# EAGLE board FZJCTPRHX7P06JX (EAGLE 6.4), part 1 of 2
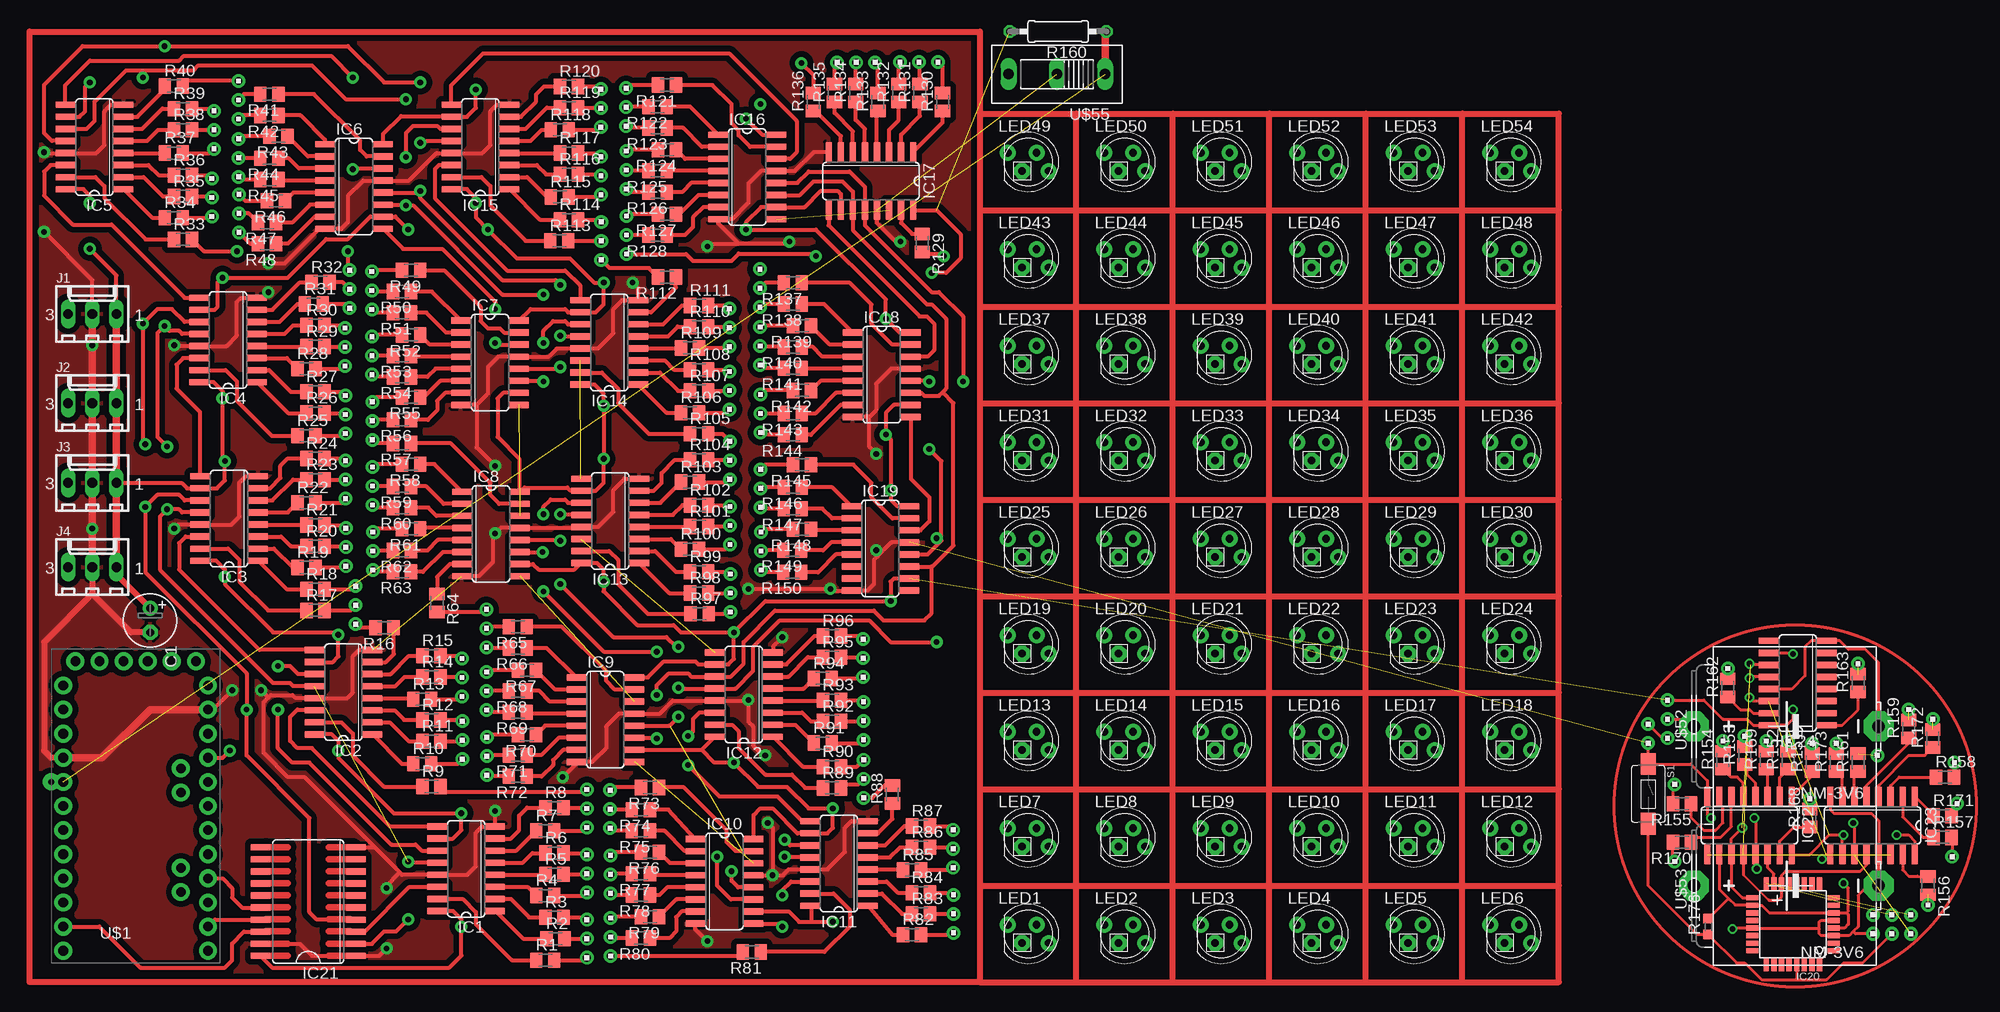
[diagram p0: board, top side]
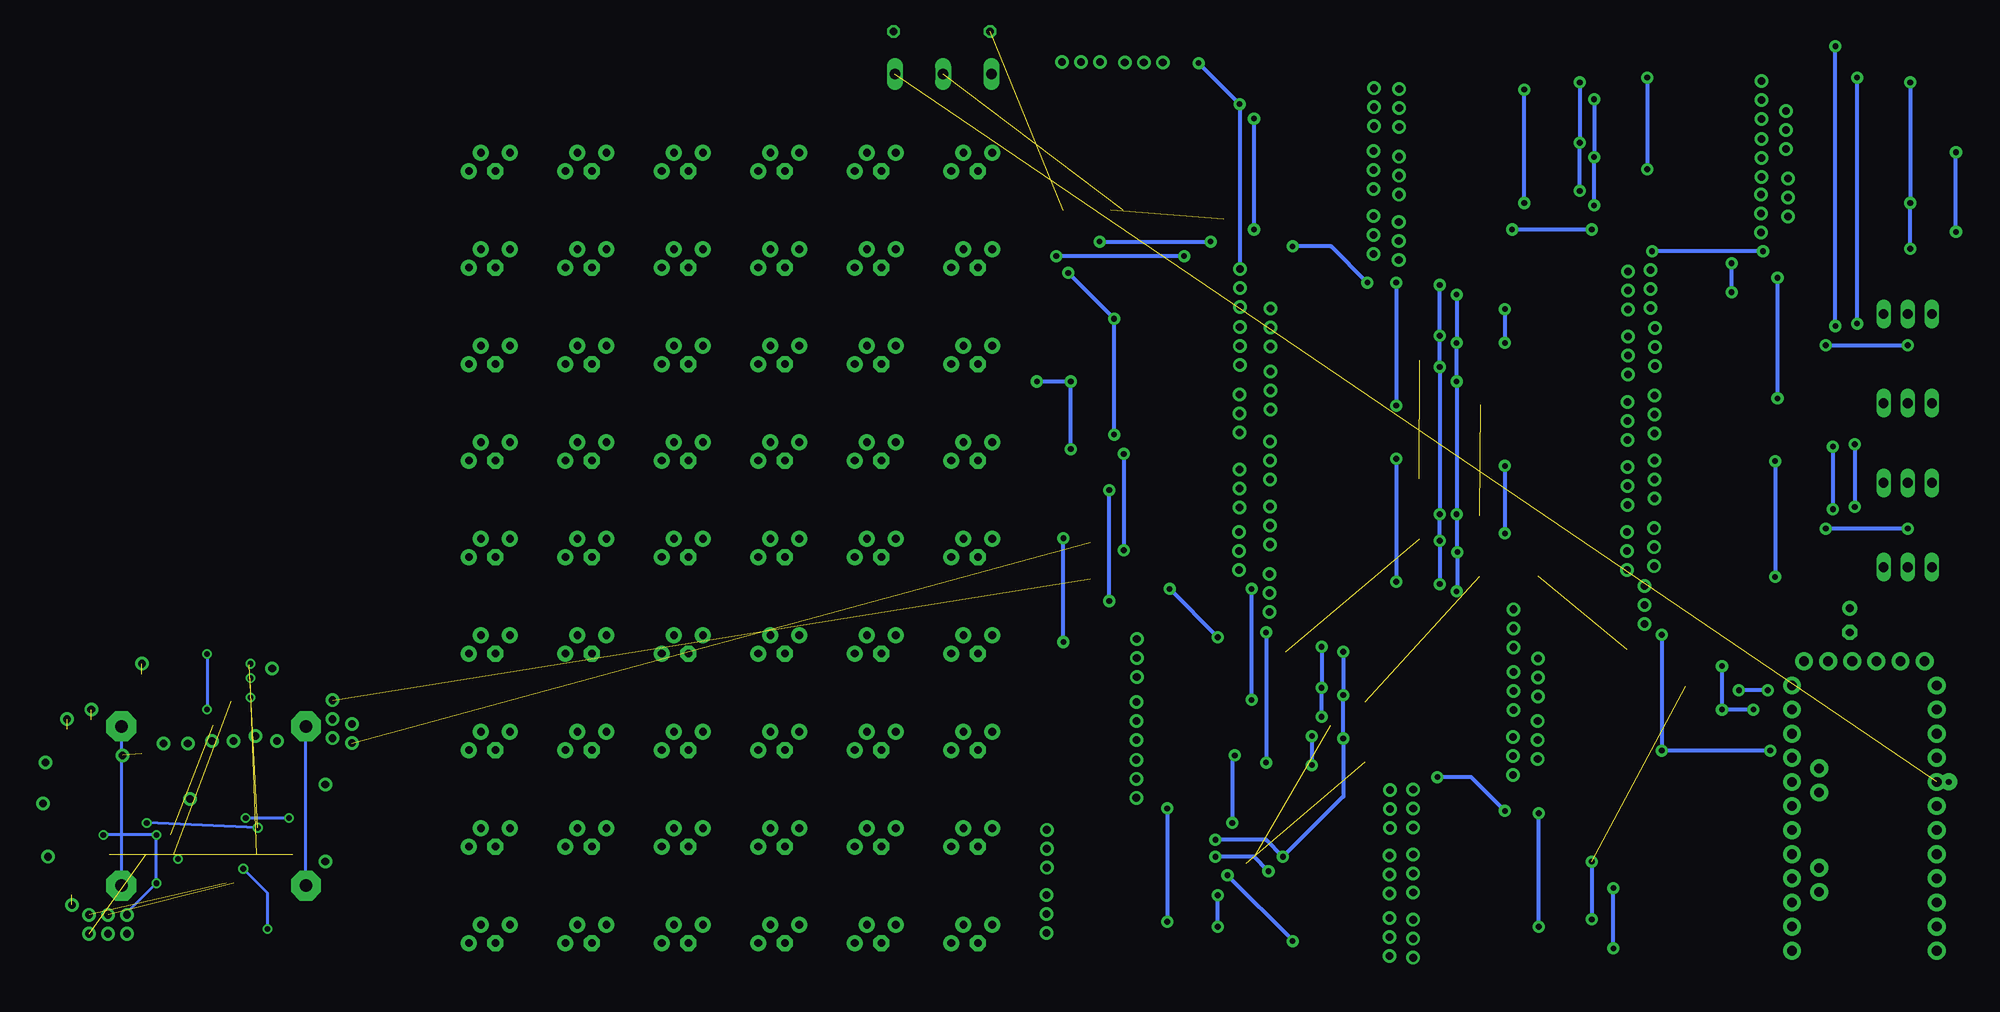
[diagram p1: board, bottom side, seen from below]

No outline drawn. Coordinates in mm, seen from the top.
Copper layers (1*16): Top 0.035mm / dielectric 1.5mm / Bottom 0.035mm
Design rules "default": minimum track width 10mil, minimum drill 24mil, track to track 8mil, track to pad 8mil, pad to pad 8mil, via to via 8mil, smd to smd 8mil, copper to edge 40mil, drill to drill 8mil, minimum pad ring 10mil, minimum via ring 8mil, stop-mask expansion 4mil, vias tented up to drill 0mil, thermal gap 10mil

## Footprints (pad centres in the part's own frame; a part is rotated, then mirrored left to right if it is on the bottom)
E2,5-6 = drill 0.813 pad 1.6: + -1.27,0 | drill 0.813 pad 1.6 octagon: - 1.27,0
SO16 = smd 0.66 x 2.032: 1 -4.445,-3.073; 2 -3.175,-3.073; 3 -1.905,-3.073; 4 -0.635,-3.073; 5 0.635,-3.073; 6 1.905,-3.073; 7 3.175,-3.073; 8 4.445,-3.073; 9 4.445,3.073; 10 3.175,3.073; 11 1.905,3.073; 12 0.635,3.073; 13 -0.635,3.073; 14 -1.905,3.073; 15 -3.175,3.073; 16 -4.445,3.073
TQFP32-08 = smd 1.27 x 0.559: 1 -4.293,2.8; 2 -4.293,2; 3 -4.293,1.2; 4 -4.293,0.4; 5 -4.293,-0.4; 6 -4.293,-1.2; 7 -4.293,-2; 8 -4.293,-2.8; 17 4.293,-2.8; 18 4.293,-2; 19 4.293,-1.2; 20 4.293,-0.4; 21 4.293,0.4; 22 4.293,1.2; 23 4.293,2; 24 4.293,2.8 | smd 0.559 x 1.27: 9 -2.8,-4.293; 10 -2,-4.293; 11 -1.2,-4.293; 12 -0.4,-4.293; 13 0.4,-4.293; 14 1.2,-4.293; 15 2,-4.293; 16 2.8,-4.293; 25 2.8,4.293; 26 2,4.293; 27 1.2,4.293; 28 0.4,4.293; 29 -0.4,4.293; 30 -1.2,4.293; 31 -2,4.293; 32 -2.8,4.293
SO20W = smd 0.66 x 2.032: 1 -5.715,-5.029; 2 -4.445,-5.029; 3 -3.175,-5.029; 4 -1.905,-5.029; 5 -0.635,-5.029; 6 0.635,-5.029; 7 1.905,-5.029; 8 3.175,-5.029; 9 4.445,-5.029; 10 5.715,-5.029; 11 5.715,5.029; 12 4.445,5.029; 13 3.175,5.029; 14 1.905,5.029; 15 0.635,5.029; 16 -0.635,5.029; 17 -1.905,5.029; 18 -3.175,5.029; 19 -4.445,5.029; 20 -5.715,5.029
6410-03 = drill 1.016 long: 1 2.54,0; 2 0,0; 3 -2.54,0
LED5MMRGB = drill 0.8 pad 1.676: 1 -2.159,0.968; 3 0.889,0.968; 4 2.159,-0.968 | drill 0.8 pad 1.676 octagon: 2 -0.635,-0.968
M0805 = smd 1.3 x 1.6: 1 -0.95,0; 2 0.95,0
0207/10 = drill 0.813 octagon: 1 -5.08,0; 2 5.08,0
R0603 = smd 1 x 1.1: 1 -0.85,0; 2 0.85,0
TACTILE-SWITCH-1101NE = smd 2.3 x 1.6: P$1 -3.15,0; P$2 3.15,0
ARDUINO_PRO_MINI = drill 1.016 pad 1.88: 1 -7.62,12.7; 2 -7.62,10.16; 3 -7.62,7.62; 4 -7.62,5.08; 5 -7.62,2.54; 6 -7.62,0; 7 -7.62,-2.54; 8 -7.62,-5.08; 9 -7.62,-7.62; 10 -7.62,-10.16; 11 -7.62,-12.7; 12 -7.62,-15.24; 13 7.62,-15.24; 14 7.62,-12.7; 15 7.62,-10.16; 16 7.62,-7.62; 17 7.62,-5.08; 18 7.62,-2.54; 19 7.62,0; 20 7.62,2.54; 21 7.62,5.08; 22 7.62,7.62; 23 7.62,10.16; 24 7.62,12.7; A4 4.763,1.429; A5 4.763,3.969; A6 4.763,-9.049; A7 4.763,-6.509; BLK -6.35,15.24; GND -3.81,15.24; GRN 6.35,15.24; RXI 1.27,15.24; TXO 3.81,15.24; VCC -1.27,15.24
1X3 = drill 0.8 pad 1.422: 1 -2,0; 2 0,0; 3 2,0
3.6V-NIMH-BATTERY = drill 1.321 pad 3.15 octagon: + -10.16,0; - 9.271,0
1X1 = drill 0.8 pad 1.422: 1 0,0
LIMIT-SWITCH = drill 1.118 long: 1 -5.08,0; 2 0,0; 3 5.08,0
2X3 = drill 0.8 pad 1.422: 1 -2,-1; 2 -2,1; 3 0,-1; 4 0,1; 5 2,-1; 6 2,1
1X2 = drill 0.8 pad 1.422: 1 -1,0; 2 1,0

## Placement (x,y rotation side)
C1  100uF  [E2,5-6]  12.7,38.1 270 top
IC1  74HC595D  [SO16]  45.97,11.94 90 top
IC2  74HC595D  [SO16]  33.05,30.53 90 top
IC3  74HC595D  [SO16]  21.01,48.82 90 top
IC4  74HC595D  [SO16]  20.9,67.61 90 top
IC5  74HC595D  [SO16]  6.83,87.93 90 top
IC6  74HC595D  [SO16]  34.16,83.77 270 top
IC7  74HC595D  [SO16]  48.49,65.23 270 top
IC8  74HC595D  [SO16]  48.59,47.19 270 top
IC9  74HC595D  [SO16]  60.63,27.64 270 top
IC10  74HC595D  [SO16]  73.18,10.62 270 top
IC11  74HC595D  [SO16]  85.22,12.5 90 top
IC12  74HC595D  [SO16]  75.21,30.28 90 top
IC13  74HC595D  [SO16]  61.14,48.56 90 top
IC14  74HC595D  [SO16]  61.04,67.36 90 top
IC15  74HC595D  [SO16]  47.47,87.93 90 top
IC16  74HC595D  [SO16]  75.56,84.79 270 top
IC17  74HC595D  [SO16]  88.6,84.35 180 top
IC18  74HC595D  [SO16]  89.74,63.96 270 top
IC19  74HC595D  [SO16]  89.59,45.67 270 top
IC20  MEGA8-AI  [TQFP32-08]  185.67,6.1 180 top
IC21  74LS245DW  [SO20W]  29.34,8.48 90 top
IC22  74HC595D  [SO16]  181.1,16.51 180 top
IC23  74HC595D  [SO16]  194.06,16.51 180 top
IC24  74HC595D  [SO16]  186.18,31.5 90 top
J1  22-27-2031-03  [6410-03]  6.6,70.36 0 top
J2  22-27-2031-03  [6410-03]  6.6,60.96 0 top
J3  22-27-2031-03  [6410-03]  6.6,52.58 0 top
J4  22-27-2031-03  [6410-03]  6.6,43.69 0 top
LED1  RGBLED_CA-5MM  [LED5MMRGB]  105.16,5.08 0 top
LED2  RGBLED_CA-5MM  [LED5MMRGB]  115.32,5.08 0 top
LED3  RGBLED_CA-5MM  [LED5MMRGB]  125.48,5.08 0 top
LED4  RGBLED_CA-5MM  [LED5MMRGB]  135.64,5.08 0 top
LED5  RGBLED_CA-5MM  [LED5MMRGB]  145.8,5.08 0 top
LED6  RGBLED_CA-5MM  [LED5MMRGB]  155.96,5.08 0 top
LED7  RGBLED_CA-5MM  [LED5MMRGB]  105.16,15.24 0 top
LED8  RGBLED_CA-5MM  [LED5MMRGB]  115.32,15.24 0 top
LED9  RGBLED_CA-5MM  [LED5MMRGB]  125.48,15.24 0 top
LED10  RGBLED_CA-5MM  [LED5MMRGB]  135.64,15.24 0 top
LED11  RGBLED_CA-5MM  [LED5MMRGB]  145.8,15.24 0 top
LED12  RGBLED_CA-5MM  [LED5MMRGB]  155.96,15.24 0 top
LED13  RGBLED_CA-5MM  [LED5MMRGB]  105.16,25.4 0 top
LED14  RGBLED_CA-5MM  [LED5MMRGB]  115.32,25.4 0 top
LED15  RGBLED_CA-5MM  [LED5MMRGB]  125.48,25.4 0 top
LED16  RGBLED_CA-5MM  [LED5MMRGB]  135.64,25.4 0 top
LED17  RGBLED_CA-5MM  [LED5MMRGB]  145.8,25.4 0 top
LED18  RGBLED_CA-5MM  [LED5MMRGB]  155.96,25.4 0 top
LED19  RGBLED_CA-5MM  [LED5MMRGB]  105.16,35.56 0 top
LED20  RGBLED_CA-5MM  [LED5MMRGB]  115.32,35.56 0 top
LED21  RGBLED_CA-5MM  [LED5MMRGB]  125.48,35.56 0 top
LED22  RGBLED_CA-5MM  [LED5MMRGB]  135.64,35.56 0 top
LED23  RGBLED_CA-5MM  [LED5MMRGB]  145.8,35.56 0 top
LED24  RGBLED_CA-5MM  [LED5MMRGB]  155.96,35.56 0 top
LED25  RGBLED_CA-5MM  [LED5MMRGB]  105.16,45.72 0 top
LED26  RGBLED_CA-5MM  [LED5MMRGB]  115.32,45.72 0 top
LED27  RGBLED_CA-5MM  [LED5MMRGB]  125.48,45.72 0 top
LED28  RGBLED_CA-5MM  [LED5MMRGB]  135.64,45.72 0 top
LED29  RGBLED_CA-5MM  [LED5MMRGB]  145.8,45.72 0 top
LED30  RGBLED_CA-5MM  [LED5MMRGB]  155.96,45.72 0 top
LED31  RGBLED_CA-5MM  [LED5MMRGB]  105.16,55.88 0 top
LED32  RGBLED_CA-5MM  [LED5MMRGB]  115.32,55.88 0 top
LED33  RGBLED_CA-5MM  [LED5MMRGB]  125.48,55.88 0 top
LED34  RGBLED_CA-5MM  [LED5MMRGB]  135.64,55.88 0 top
LED35  RGBLED_CA-5MM  [LED5MMRGB]  145.8,55.88 0 top
LED36  RGBLED_CA-5MM  [LED5MMRGB]  155.96,55.88 0 top
LED37  RGBLED_CA-5MM  [LED5MMRGB]  105.16,66.04 0 top
LED38  RGBLED_CA-5MM  [LED5MMRGB]  115.32,66.04 0 top
LED39  RGBLED_CA-5MM  [LED5MMRGB]  125.48,66.04 0 top
LED40  RGBLED_CA-5MM  [LED5MMRGB]  135.64,66.04 0 top
LED41  RGBLED_CA-5MM  [LED5MMRGB]  145.8,66.04 0 top
LED42  RGBLED_CA-5MM  [LED5MMRGB]  155.96,66.04 0 top
LED43  RGBLED_CA-5MM  [LED5MMRGB]  105.16,76.2 0 top
LED44  RGBLED_CA-5MM  [LED5MMRGB]  115.32,76.2 0 top
LED45  RGBLED_CA-5MM  [LED5MMRGB]  125.48,76.2 0 top
LED46  RGBLED_CA-5MM  [LED5MMRGB]  135.64,76.2 0 top
LED47  RGBLED_CA-5MM  [LED5MMRGB]  145.8,76.2 0 top
LED48  RGBLED_CA-5MM  [LED5MMRGB]  155.96,76.2 0 top
LED49  RGBLED_CA-5MM  [LED5MMRGB]  105.16,86.36 0 top
LED50  RGBLED_CA-5MM  [LED5MMRGB]  115.32,86.36 0 top
LED51  RGBLED_CA-5MM  [LED5MMRGB]  125.48,86.36 0 top
LED52  RGBLED_CA-5MM  [LED5MMRGB]  135.64,86.36 0 top
LED53  RGBLED_CA-5MM  [LED5MMRGB]  145.8,86.36 0 top
LED54  RGBLED_CA-5MM  [LED5MMRGB]  155.96,86.36 0 top
R1  150  [M0805]  54.31,2.31 0 top
R2  100  [M0805]  55.37,4.57 0 top
R3  100  [M0805]  55.27,6.83 0 top
R4  150  [M0805]  54.31,9.12 0 top
R5  100  [M0805]  55.27,11.35 0 top
R6  100  [M0805]  55.27,13.59 0 top
R7  150  [M0805]  54.31,15.93 0 top
R8  100  [M0805]  55.27,18.36 0 top
R9  100  [M0805]  42.32,20.6 0 top
R10  150  [M0805]  41.35,22.99 0 top
R11  100  [M0805]  42.32,25.37 0 top
R12  100  [M0805]  42.32,27.61 0 top
R13  150  [M0805]  41.35,29.79 0 top
R14  100  [M0805]  42.32,32.13 0 top
R15  100  [M0805]  42.32,34.37 0 top
R16  150  [M0805]  37.39,37.31 180 top
R17  100  [M0805]  30.12,39.14 0 top
R18  100  [M0805]  30.12,41.38 0 top
R19  150  [M0805]  29.16,43.66 0 top
R20  100  [M0805]  30.12,45.9 0 top
R21  100  [M0805]  30.12,48.13 0 top
R22  150  [M0805]  29.16,50.47 0 top
R23  100  [M0805]  30.12,52.91 0 top
R24  100  [M0805]  30.12,55.14 0 top
R25  150  [M0805]  29.16,57.53 0 top
R26  100  [M0805]  30.12,59.92 0 top
R27  100  [M0805]  30.12,62.15 0 top
R28  150  [M0805]  29.16,64.59 0 top
R29  100  [M0805]  30.12,66.93 0 top
R30  100  [M0805]  30.12,69.16 0 top
R31  150  [M0805]  29.92,71.4 0 top
R32  100  [M0805]  30.63,73.69 0 top
R33  100  [M0805]  16.15,78.21 0 top
R34  150  [M0805]  15.19,80.49 0 top
R35  100  [M0805]  16.15,82.73 0 top
R36  100  [M0805]  16.15,84.96 0 top
R37  150  [M0805]  15.19,87.3 0 top
R38  100  [M0805]  16.15,89.74 0 top
R39  100  [M0805]  16.15,91.97 0 top
R40  150  [M0805]  15.19,94.36 0 top
R41  100  [M0805]  25.25,93.5 180 top
R42  100  [M0805]  25.25,91.26 180 top
R43  150  [M0805]  26.21,89.08 180 top
R44  100  [M0805]  25.25,86.74 180 top
R45  100  [M0805]  25.25,84.51 180 top
R46  150  [M0805]  25.96,82.27 180 top
R47  100  [M0805]  24.99,79.98 180 top
R48  100  [M0805]  24.99,77.75 180 top
R49  150  [M0805]  40.18,74.96 180 top
R50  100  [M0805]  39.22,72.72 180 top
R51  100  [M0805]  39.22,70.48 180 top
R52  150  [M0805]  40.18,68.15 180 top
R53  100  [M0805]  39.22,65.96 180 top
R54  100  [M0805]  39.22,63.73 180 top
R55  150  [M0805]  40.18,61.59 180 top
R56  100  [M0805]  39.22,59.21 180 top
R57  100  [M0805]  39.22,56.72 180 top
R58  150  [M0805]  40.18,54.53 180 top
R59  100  [M0805]  39.22,52.2 180 top
R60  100  [M0805]  39.22,49.96 180 top
R61  150  [M0805]  40.18,47.73 180 top
R62  100  [M0805]  39.22,45.44 180 top
R63  100  [M0805]  39.22,43.21 180 top
R64  150  [M0805]  42.9,39.93 270 top
R65  100  [M0805]  51.41,37.41 180 top
R66  100  [M0805]  51.41,35.18 180 top
R67  150  [M0805]  52.37,32.84 180 top
R68  100  [M0805]  51.41,30.66 180 top
R69  100  [M0805]  51.41,28.42 180 top
R70  150  [M0805]  52.37,26.04 180 top
R71  100  [M0805]  51.41,23.9 180 top
R72  100  [M0805]  51.41,21.67 180 top
R73  150  [M0805]  65.33,20.5 180 top
R74  100  [M0805]  64.36,18.16 180 top
R75  100  [M0805]  64.36,15.93 180 top
R76  150  [M0805]  65.33,13.69 180 top
R77  100  [M0805]  64.36,11.4 180 top
R78  100  [M0805]  64.36,9.17 180 top
R79  150  [M0805]  65.33,6.88 180 top
R80  100  [M0805]  64.36,4.65 180 top
R81  100  [M0805]  76.05,3.17 180 top
R82  150  [M0805]  92.91,5 0 top
R83  100  [M0805]  93.88,7.19 0 top
R84  100  [M0805]  93.88,9.42 0 top
R85  150  [M0805]  92.91,11.81 0 top
R86  100  [M0805]  93.88,14.2 0 top
R87  100  [M0805]  93.88,16.43 0 top
R88  150  [M0805]  90.86,19.76 90 top
R89  100  [M0805]  84.48,20.45 0 top
R90  100  [M0805]  84.48,22.68 0 top
R91  150  [M0805]  83.52,25.17 0 top
R92  100  [M0805]  84.48,27.46 0 top
R93  100  [M0805]  84.48,29.69 0 top
R94  150  [M0805]  83.52,31.98 0 top
R95  100  [M0805]  84.48,34.21 0 top
R96  100  [M0805]  84.48,36.45 0 top
R97  150  [M0805]  70.56,38.79 0 top
R98  100  [M0805]  70.51,40.97 0 top
R99  100  [M0805]  70.51,43.21 0 top
R100  150  [M0805]  69.55,45.59 0 top
R101  100  [M0805]  70.51,47.98 0 top
R102  100  [M0805]  70.51,50.22 0 top
R103  150  [M0805]  69.55,52.65 0 top
R104  100  [M0805]  70.51,54.99 0 top
R105  100  [M0805]  70.51,57.73 0 top
R106  150  [M0805]  69.55,59.97 0 top
R107  100  [M0805]  70.51,62.26 0 top
R108  100  [M0805]  70.51,64.49 0 top
R109  150  [M0805]  69.55,66.78 0 top
R110  100  [M0805]  70.51,69.01 0 top
R111  100  [M0805]  70.51,71.25 0 top
R112  150  [M0805]  67.11,74.24 180 top
R113  100  [M0805]  55.78,78.05 0 top
R114  100  [M0805]  56.79,80.29 0 top
R115  150  [M0805]  55.83,82.68 0 top
R116  100  [M0805]  56.79,85.06 0 top
R117  100  [M0805]  56.79,87.3 0 top
R118  150  [M0805]  55.83,89.74 0 top
R119  100  [M0805]  56.79,92.08 0 top
R120  100  [M0805]  56.79,94.31 0 top
R121  150  [M0805]  67.11,94.46 180 top
R122  100  [M0805]  66.14,92.18 180 top
R123  100  [M0805]  66.14,89.94 180 top
R124  150  [M0805]  67.11,87.66 180 top
R125  100  [M0805]  66.14,85.42 180 top
R126  100  [M0805]  66.14,83.19 180 top
R127  150  [M0805]  67.11,80.85 180 top
R128  100  [M0805]  66.14,78.66 180 top
R129  100  [M0805]  94.01,77.83 270 top
R130  150  [M0805]  96.14,92.66 90 top
R131  100  [M0805]  93.75,93.62 90 top
R132  100  [M0805]  91.52,93.62 90 top
R133  150  [M0805]  89.33,92.66 90 top
R134  100  [M0805]  87,93.62 90 top
R135  100  [M0805]  84.76,93.62 90 top
R136  150  [M0805]  82.52,92.66 90 top
R137  100  [M0805]  80.37,73.63 180 top
R138  100  [M0805]  80.37,71.4 180 top
R139  150  [M0805]  81.33,69.11 180 top
R140  100  [M0805]  80.37,66.88 180 top
R141  100  [M0805]  80.37,64.64 180 top
R142  150  [M0805]  81.33,62.31 180 top
R143  100  [M0805]  80.37,59.87 180 top
R144  100  [M0805]  80.37,57.63 180 top
R145  150  [M0805]  81.33,54.48 180 top
R146  100  [M0805]  80.37,52.1 180 top
R147  100  [M0805]  80.37,49.86 180 top
R148  150  [M0805]  81.33,47.68 180 top
R149  100  [M0805]  80.31,45.49 180 top
R150  100  [M0805]  80.31,43.15 180 top
R151  100  [M0805]  187.71,23.11 90 top
R152  100  [M0805]  185.17,23.37 90 top
R153  100  [M0805]  180.59,23.88 90 top
R154  100  [M0805]  178.31,23.37 90 top
R155  100  [M0805]  173.99,18.8 180 top
R156  100  [M0805]  199.9,10.16 270 top
R157  100  [M0805]  201.42,15.24 0 top
R158  100  [M0805]  201.68,21.59 0 top
R159  100  [M0805]  197.87,26.67 90 top
R160  10K  [0207/10]  108.31,100.1 180 top
R161  100  [M0805]  192.53,23.11 90 top
R162  100  [M0805]  178.82,30.99 90 top
R163  100  [M0805]  192.53,31.5 90 top
R168  150  [M0805]  187.45,17.27 90 top
R169  150  [M0805]  182.88,23.37 90 top
R170  150  [M0805]  173.99,14.73 180 top
R171  150  [M0805]  201.42,17.53 0 top
R172  150  [M0805]  200.41,25.65 90 top
R173  150  [M0805]  190.25,23.11 90 top
R176  10K  [R0603]  176.78,5.84 90 top
S1  SWITCH-MOMENTARY-2-SMD-1101NE  [TACTILE-SWITCH-1101NE]  170.43,19.81 270 top
U$1  ARDUINO_PRO_MINI  [ARDUINO_PRO_MINI]  11.18,18.54 0 top
U$2  1X3  [1X3]  58.67,4.57 270 top
U$3  1X3  [1X3]  58.67,11.43 270 top
U$4  1X3  [1X3]  58.67,18.29 270 top
U$5  1X3  [1X3]  45.57,25.48 270 top
U$6  1X3  [1X3]  45.54,32.08 270 top
U$7  1X3  [1X3]  34.34,39.7 270 top
U$8  1X3  [1X3]  33.3,45.8 270 top
U$9  1X3  [1X3]  33.27,52.91 270 top
U$10  1X3  [1X3]  33.25,59.77 270 top
U$11  1X3  [1X3]  33.22,66.88 270 top
U$12  1X3  [1X3]  33.71,72.97 270 top
U$13  1X3  [1X3]  19.2,82.63 270 top
U$14  1X3  [1X3]  19.43,89.74 270 top
U$15  1X3  [1X3]  22,92.89 90 top
U$16  1X3  [1X3]  22.02,86.79 90 top
U$17  1X3  [1X3]  22.05,80.95 90 top
U$18  1X3  [1X3]  36.04,72.82 90 top
U$19  1X3  [1X3]  36.07,65.96 90 top
U$20  1X3  [1X3]  36.09,59.11 90 top
U$21  1X3  [1X3]  36.12,52.25 90 top
U$22  1X3  [1X3]  36.14,45.39 90 top
U$23  1X3  [1X3]  48.11,37.26 90 top
U$24  1X3  [1X3]  48.13,30.66 90 top
U$25  1X3  [1X3]  48.16,23.8 90 top
U$26  1X3  [1X3]  61.14,18.21 90 top
U$27  1X3  [1X3]  61.16,11.35 90 top
U$28  1X3  [1X3]  61.19,4.75 90 top
U$29  1X3  [1X3]  97.28,7.19 270 top
U$30  1X3  [1X3]  97.26,14.05 270 top
U$31  1X3  [1X3]  87.83,21.41 270 top
U$32  1X3  [1X3]  87.81,27.51 270 top
U$33  1X3  [1X3]  87.78,34.11 270 top
U$34  1X3  [1X3]  73.79,40.97 270 top
U$35  1X3  [1X3]  73.76,48.08 270 top
U$36  1X3  [1X3]  73.74,54.94 270 top
U$37  1X3  [1X3]  73.71,62.31 270 top
U$38  1X3  [1X3]  73.69,68.91 270 top
U$39  1X3  [1X3]  60.2,78.05 270 top
U$40  1X3  [1X3]  60.17,84.91 270 top
U$41  1X3  [1X3]  60.15,92.02 270 top
U$42  1X3  [1X3]  62.81,92.13 90 top
U$43  1X3  [1X3]  62.84,85.52 90 top
U$44  1X3  [1X3]  62.87,78.66 90 top
U$45  1X3  [1X3]  93.65,96.88 0 top
U$46  1X3  [1X3]  87.05,96.85 0 top
U$47  1X3  [1X3]  76.91,73.08 90 top
U$48  1X3  [1X3]  76.94,66.98 90 top
U$49  1X3  [1X3]  76.96,59.87 90 top
U$50  1X3  [1X3]  76.99,51.99 90 top
U$51  1X3  [1X3]  77.01,45.39 90 top
U$52  3.6V-NIMH-BATTERY  [3.6V-NIMH-BATTERY]  185.42,26.92 0 top
U$53  3.6V-NIMH-BATTERY  [3.6V-NIMH-BATTERY]  185.42,10.16 0 top
U$54  1X1  [1X1]  187.45,19.3 0 top
U$55  LIMIT-SWITCH  [LIMIT-SWITCH]  108.18,95.61 180 top
U$56  1X1  [1X1]  187.71,25.15 0 top
U$57  1X1  [1X1]  185.17,25.4 0 top
U$58  1X1  [1X1]  182.88,25.4 0 top
U$59  1X1  [1X1]  180.59,25.91 0 top
U$60  1X1  [1X1]  178.31,25.4 0 top
U$61  1X1  [1X1]  173.23,12.7 0 top
U$62  1X1  [1X1]  173.23,20.83 0 top
U$63  2X3  [2X3]  196.09,6.1 0 top
U$64  1X3  [1X3]  172.47,27.69 90 top
U$65  1X1  [1X1]  199.9,8.13 0 top
U$66  1X1  [1X1]  202.95,18.8 0 top
U$67  1X1  [1X1]  202.44,13.21 0 top
U$68  1X1  [1X1]  202.69,23.11 0 top
U$69  1X1  [1X1]  200.41,27.69 0 top
U$70  1X1  [1X1]  197.87,28.7 0 top
U$71  1X1  [1X1]  194.56,23.88 0 top
U$72  1X1  [1X1]  190.25,25.15 0 top
U$73  1X1  [1X1]  178.82,33.02 0 top
U$74  1X1  [1X1]  192.53,33.53 0 top
U$75  1X2  [1X2]  170.43,26.16 90 top

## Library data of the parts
C1 R1-R163 R168-R173 R176 = resistor
IC1-IC19 IC22-IC24 = 74xx-eu
IC20 = atmel; MPN: ATMEGA8-16AU; OC_FARNELL: 9171371; OC_NEWARK: 73M8863
IC21 = 74xx-us
J1-J4 = con-molex; OC_FARNELL: unknown; OC_NEWARK: unknown
LED1-LED54 = adafruit
S1 = SparkFun-Electromechanical
U$1 = SparkFun-Boards
U$2-U$51 U$54 U$56-U$75 = headers(2mm)
U$52 U$53 U$55 = ggaqquay

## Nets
CLOCK: IC1.11 IC2.11 IC3.11 IC4.11 IC5.11 IC6.11 IC7.11 IC8.11 IC9.11 IC10.11 IC11.11 IC12.11 IC13.11 IC14.11 IC15.11 IC16.11 IC17.11 IC18.11 IC19.11 IC21.4
CLOCK2: IC20.17 IC22.11 IC23.11 IC24.11 U$63.5
D8: IC21.18 U$1.11
D11: IC21.17 U$1.14
D13: IC21.16 U$1.16
DATA: IC1.14 IC21.3
DATA2: IC20.15 IC22.14 U$63.6
GND: C1.- IC1.8 IC1.13 IC2.8 IC2.13 IC3.8 IC3.13 IC4.8 IC4.13 IC5.8 IC5.13 IC6.8 IC6.13 IC7.8 IC7.13 IC8.8 IC8.13 IC9.8 IC9.13 IC10.8 IC10.13 IC11.8 IC11.13 IC12.8 IC12.13 IC13.8 IC13.13 IC14.8 IC14.13 IC15.8 IC15.13 IC16.8 IC16.13 IC17.8 IC17.13 IC18.8 IC18.13 IC19.8 IC19.13 IC20.3 IC20.5 IC20.21 IC21.1 IC21.10 IC21.19 IC22.8 IC22.13 IC23.8 IC23.13 IC24.8 IC24.13 J1.2 J2.2 J3.2 J4.2 S1.P$1 U$1.4 U$1.23 U$52.- U$53.- U$55.2 U$63.1 U$75.1
LATCH: IC1.12 IC2.12 IC3.12 IC4.12 IC5.12 IC6.12 IC7.12 IC8.12 IC9.12 IC10.12 IC11.12 IC12.12 IC13.12 IC14.12 IC15.12 IC16.12 IC17.12 IC18.12 IC19.12 IC21.2
LATCH2: IC20.14 IC22.12 IC23.12 IC24.12
MISO: IC20.16 U$63.4
N$1: R160.1 U$1.5 U$55.1
N$4: IC22.15 R168.1
N$5: R81.2 U$28.1
N$6: IC10.9 IC11.14
N$7: IC22.1 R151.1
N$8: IC22.2 R152.1
N$9: R168.2 U$54.1
N$10: R151.2 U$56.1
N$11: R152.2 U$57.1
N$12: R169.2 U$58.1
N$13: R153.2 U$59.1
N$14: R154.2 U$60.1
N$15: R170.2 U$61.1
N$16: R155.2 U$62.1
N$17: IC22.3 R169.1
N$18: IC22.4 R153.1
N$19: IC22.5 R154.1
N$20: IC22.6 R170.1
N$21: IC22.7 R155.1
N$22: IC23.15 R156.1
N$23: R156.2 U$65.1
N$24: R171.2 U$66.1
N$25: R157.2 U$67.1
N$26: R158.2 U$68.1
N$27: R172.2 U$69.1
N$28: R159.2 U$70.1
N$29: IC1.15 R1.1
N$30: IC1.1 R2.1
N$31: IC1.2 R3.1
N$32: R1.2 U$2.3
N$33: R2.2 U$2.2
N$34: R3.2 U$2.1
N$35: R4.2 U$3.3
N$36: R5.2 U$3.2
N$37: R6.2 U$3.1
N$38: R7.2 U$4.3
N$39: R8.2 U$4.2
N$40: IC1.3 R4.1
N$41: IC1.4 R5.1
N$42: IC1.5 R6.1
N$43: IC1.6 R7.1
N$44: IC1.7 R8.1
N$45: IC2.15 R9.1
N$46: R9.2 U$4.1
N$47: R10.2 U$5.3
N$48: R11.2 U$5.2
N$49: R12.2 U$5.1
N$50: R13.2 U$6.3
N$51: R14.2 U$6.2
N$52: R15.2 U$6.1
N$53: R16.2 U$7.3
N$54: R17.2 U$7.2
N$55: R18.2 U$7.1
N$56: R19.2 U$8.3
N$57: R20.2 U$8.2
N$58: R21.2 U$8.1
N$59: R22.2 U$9.3
N$60: R23.2 U$9.2
N$61: R24.2 U$9.1
N$62: R25.2 U$10.3
N$63: R26.2 U$10.2
N$64: R27.2 U$10.1
N$65: R28.2 U$11.3
N$66: R29.2 U$11.2
N$67: R30.2 U$11.1
N$68: R31.2 U$12.3
N$69: R32.2 U$12.2
N$70: R33.2 U$12.1
N$71: R34.2 U$13.3
N$72: R35.2 U$13.2
N$73: R36.2 U$13.1
N$74: R37.2 U$14.3
N$75: R38.2 U$14.2
N$76: R39.2 U$14.1
N$77: R40.2 U$15.3
N$78: R41.2 U$15.2
N$79: R42.2 U$15.1
N$80: R43.2 U$16.3
N$81: R44.2 U$16.2
N$82: R45.2 U$16.1
N$83: R46.2 U$17.3
N$84: R47.2 U$17.2
N$85: R48.2 U$17.1
N$86: R49.2 U$18.3
N$87: R50.2 U$18.2
N$88: R51.2 U$18.1
N$89: R52.2 U$19.3
N$90: R53.2 U$19.2
N$91: R54.2 U$19.1
N$92: R55.2 U$20.3
N$93: R56.2 U$20.2
N$94: R57.2 U$20.1
N$95: R58.2 U$21.3
N$96: R59.2 U$21.2
N$97: R60.2 U$21.1
N$98: R61.2 U$22.3
N$99: R62.2 U$22.2
N$100: R63.2 U$22.1
N$101: R64.2 U$23.3
N$102: R65.2 U$23.2
N$103: R66.2 U$23.1
N$104: R67.2 U$24.3
N$105: R68.2 U$24.2
N$106: R69.2 U$24.1
N$107: R70.2 U$25.3
N$108: R71.2 U$25.2
N$109: R72.2 U$25.1
N$110: R73.2 U$26.3
N$111: R74.2 U$26.2
N$112: R75.2 U$26.1
N$113: R76.2 U$27.3
N$114: R77.2 U$27.2
N$115: R78.2 U$27.1
N$116: R79.2 U$28.3
N$117: R80.2 U$28.2
N$118: R82.2 U$29.3
N$119: R83.2 U$29.2
N$120: R84.2 U$29.1
N$121: R85.2 U$30.3
N$122: R86.2 U$30.2
N$123: R87.2 U$30.1
N$124: R88.2 U$31.3
N$125: R89.2 U$31.2
N$126: R90.2 U$31.1
N$127: R91.2 U$32.3
N$128: R92.2 U$32.2
N$129: R93.2 U$32.1
N$130: R94.2 U$33.3
N$131: R95.2 U$33.2
N$132: R96.2 U$33.1
N$133: R97.2 U$34.3
N$134: R98.2 U$34.2
N$135: R99.2 U$34.1
N$136: R100.2 U$35.3
N$137: R101.2 U$35.2
N$138: R102.2 U$35.1
N$139: R103.2 U$36.3
N$140: R104.2 U$36.2
N$141: R105.2 U$36.1
N$142: R106.2 U$37.3
N$143: R107.2 U$37.2
N$144: R108.2 U$37.1
N$145: R109.2 U$38.3
N$146: R110.2 U$38.2
N$147: R111.2 U$38.1
N$148: R112.2 U$39.3
N$149: R113.2 U$39.2
N$150: R114.2 U$39.1
N$151: R115.2 U$40.3
N$152: R116.2 U$40.2
N$153: R117.2 U$40.1
N$154: R118.2 U$41.3
N$155: R119.2 U$41.2
N$156: R120.2 U$41.1
N$157: R121.2 U$42.3
N$158: R122.2 U$42.2
N$159: R123.2 U$42.1
N$160: R124.2 U$43.3
N$161: R125.2 U$43.2
N$162: R126.2 U$43.1
N$163: R127.2 U$44.3
N$164: R128.2 U$44.2
N$165: R129.2 U$44.1
N$166: R130.2 U$45.3
N$167: R131.2 U$45.2
N$168: R132.2 U$45.1
N$169: R133.2 U$46.3
N$170: R134.2 U$46.2
N$171: R135.2 U$46.1
N$172: R136.2 U$47.3
N$173: R137.2 U$47.2
N$174: R138.2 U$47.1
N$175: R139.2 U$48.3
N$176: R140.2 U$48.2
N$177: R141.2 U$48.1
N$178: R142.2 U$49.3
N$179: R143.2 U$49.2
N$180: R144.2 U$49.1
N$181: R145.2 U$50.3
N$182: R146.2 U$50.2
N$183: R147.2 U$50.1
N$184: R148.2 U$51.3
N$185: R149.2 U$51.2
N$186: R150.2 U$51.1
N$187: R161.2 U$71.1
N$188: R173.2 U$72.1
N$189: R162.2 U$73.1
N$190: R163.2 U$74.1
N$196: IC11.15 R81.1
N$197: IC11.1 R82.1
N$198: IC11.2 R83.1
N$199: IC11.3 R84.1
N$200: IC11.4 R85.1
N$201: IC11.5 R86.1
N$202: IC11.6 R87.1
N$203: IC11.7 R88.1
N$204: IC12.15 R89.1
N$205: IC12.1 R90.1
N$206: IC12.2 R91.1
N$207: IC12.3 R92.1
N$208: IC12.4 R93.1
N$209: IC12.5 R94.1
N$210: IC12.6 R95.1
N$211: IC12.7 R96.1
N$212: IC13.15 R97.1
N$213: IC13.1 R98.1
N$214: IC13.2 R99.1
N$215: IC13.3 R100.1
N$216: IC13.4 R101.1
N$217: IC13.5 R102.1
N$218: IC13.6 R103.1
N$219: IC13.7 R104.1
N$220: IC14.15 R105.1
N$221: IC14.1 R106.1
N$222: IC14.2 R107.1
N$223: IC14.3 R108.1
N$224: IC14.4 R109.1
N$225: IC14.5 R110.1
N$226: IC14.6 R111.1
N$227: IC14.7 R112.1
N$228: IC15.15 R113.1
N$229: IC15.1 R114.1
N$230: IC15.2 R115.1
N$231: IC15.3 R116.1
N$232: IC15.4 R117.1
N$233: IC15.5 R118.1
N$234: IC15.6 R119.1
N$235: IC15.7 R120.1
N$236: IC16.15 R121.1
N$237: IC16.1 R122.1
N$238: IC16.2 R123.1
N$239: IC16.3 R124.1
N$240: IC16.4 R125.1
N$241: IC16.5 R126.1
N$242: IC16.6 R127.1
N$243: IC16.7 R128.1
N$244: IC17.15 R129.1
N$245: IC17.1 R130.1
N$246: IC17.2 R131.1
N$247: IC17.3 R132.1
N$248: IC17.4 R133.1
N$249: IC17.5 R134.1
N$250: IC17.6 R135.1
N$251: IC17.7 R136.1
N$252: IC18.15 R137.1
N$253: IC18.1 R138.1
N$254: IC18.2 R139.1
N$255: IC18.3 R140.1
N$256: IC18.4 R141.1
N$257: IC18.5 R142.1
N$258: IC18.6 R143.1
N$259: IC18.7 R144.1
N$260: IC19.15 R145.1
N$261: IC19.1 R146.1
N$262: IC19.2 R147.1
N$263: IC19.3 R148.1
N$264: IC19.4 R149.1
N$265: IC19.5 R150.1
N$273: IC24.1 R163.1
N$274: IC24.15 R162.1
N$275: IC23.7 R173.1
N$276: IC10.7 R80.1
N$277: IC10.6 R79.1
N$278: IC10.5 R78.1
N$279: IC10.4 R77.1
N$280: IC10.3 R76.1
N$281: IC10.2 R75.1
N$282: IC10.1 R74.1
N$283: IC10.15 R73.1
N$284: IC9.7 R72.1
N$285: IC9.6 R71.1
N$286: IC9.5 R70.1
N$287: IC9.4 R69.1
N$288: IC9.3 R68.1
N$289: IC9.2 R67.1
N$290: IC9.1 R66.1
N$291: IC9.15 R65.1
N$292: IC8.7 R64.1
N$293: IC8.6 R63.1
N$294: IC8.5 R62.1
N$295: IC8.4 R61.1
N$296: IC8.3 R60.1
N$297: IC8.2 R59.1
N$298: IC8.1 R58.1
N$299: IC8.15 R57.1
N$300: IC7.7 R56.1
N$301: IC7.6 R55.1
N$302: IC7.5 R54.1
N$303: IC7.4 R53.1
N$304: IC7.3 R52.1
N$305: IC7.2 R51.1
N$306: IC7.1 R50.1
N$307: IC7.15 R49.1
N$308: IC6.7 R48.1
N$309: IC6.6 R47.1
N$310: IC6.5 R46.1
N$311: IC6.4 R45.1
N$312: IC6.3 R44.1
N$313: IC6.2 R43.1
N$314: IC6.1 R42.1
N$315: IC6.15 R41.1
N$316: IC5.7 R40.1
N$317: IC5.6 R39.1
N$318: IC5.5 R38.1
N$319: IC5.4 R37.1
N$320: IC5.3 R36.1
N$321: IC5.2 R35.1
N$322: IC5.1 R34.1
N$323: IC5.15 R33.1
N$324: IC4.7 R32.1
N$325: IC4.6 R31.1
N$326: IC4.5 R30.1
N$327: IC4.4 R29.1
N$328: IC4.3 R28.1
N$329: IC4.2 R27.1
N$330: IC4.1 R26.1
N$331: IC4.15 R25.1
N$332: IC3.7 R24.1
N$333: IC3.6 R23.1
N$334: IC3.5 R22.1
N$335: IC3.4 R21.1
N$336: IC3.3 R20.1
N$337: IC3.2 R19.1
N$338: IC3.1 R18.1
N$339: IC3.15 R17.1
N$340: IC2.7 R16.1
N$341: IC2.6 R15.1
N$342: IC2.5 R14.1
N$343: IC2.4 R13.1
N$344: IC2.3 R12.1
N$345: IC2.2 R11.1
N$346: IC2.1 R10.1
N$347: IC2.9 IC3.14
N$348: IC1.9 IC2.14
N$349: IC3.9 IC4.14
N$350: IC4.9 IC5.14
N$351: IC5.9 IC6.14
N$352: IC6.9 IC7.14
N$353: IC7.9 IC8.14
N$354: IC8.9 IC9.14
N$355: IC9.9 IC10.14
N$356: IC11.9 IC12.14
N$357: IC12.9 IC13.14
N$358: IC13.9 IC14.14
N$359: IC14.9 IC15.14
N$360: IC15.9 IC16.14
N$361: IC16.9 IC17.14
N$362: IC17.9 IC18.14
N$363: IC18.9 IC19.14
N$364: IC23.6 R161.1
N$365: IC23.5 R159.1
N$366: IC23.4 R172.1
N$367: IC23.3 R158.1
N$368: IC23.2 R157.1
N$369: IC23.1 R171.1
N$370: IC23.9 IC24.14
N$371: IC22.9 IC23.14
N$374: U$64.1 U$75.2
N$375: U$52.+ U$53.+ U$64.2
RESET2: IC20.29 R176.1 S1.P$2 U$63.3
VCC: C1.+ IC1.10 IC1.16 IC2.10 IC2.16 IC3.10 IC3.16 IC4.10 IC4.16 IC5.10 IC5.16 IC6.10 IC6.16 IC7.10 IC7.16 IC8.10 IC8.16 IC9.10 IC9.16 IC10.10 IC10.16 IC11.10 IC11.16 IC12.10 IC12.16 IC13.10 IC13.16 IC14.10 IC14.16 IC15.10 IC15.16 IC16.10 IC16.16 IC17.10 IC17.16 IC18.10 IC18.16 IC19.10 IC19.16 IC20.4 IC20.6 IC20.18 IC21.20 IC22.10 IC22.16 IC23.10 IC23.16 IC24.10 IC24.16 J1.1 J2.1 J3.1 J4.1 R160.2 R176.2 U$1.21 U$63.2 U$64.3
